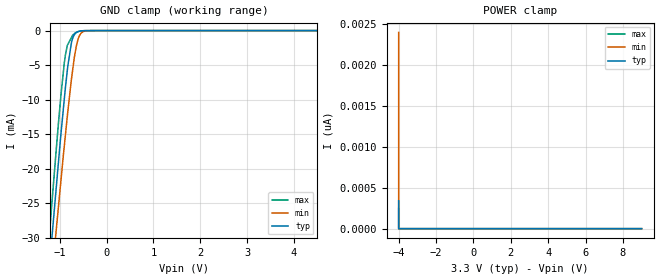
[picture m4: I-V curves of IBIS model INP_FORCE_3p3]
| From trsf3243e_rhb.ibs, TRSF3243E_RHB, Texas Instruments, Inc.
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[Model]   INP_FORCE_3p3
Model_type   Input
Vinl = 0.6
Vinh = 2.4
|   typ   min   max
C_comp   0.802pF	0.773pF	0.843pF
[Voltage Range]   3.3   3   3.6
[Temperature Range]   27   110   -40
[Power Clamp Reference]   3.3   3   3.6
[GND Clamp Reference]   0   0   0
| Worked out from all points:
|   GND clamp passes 1 mA (typ) near -0.72 V on its own axis
[GND Clamp]
|   Voltage   I(typ)   I(min)   I(max)
-4V       -268.4mA   -254.7mA   -282.4mA
-1.226V   -34.73mA   -40.07mA   -30.27mA
-1.166V   -30.07mA   -35.67mA   -25.03mA
-1.121V   -26.57mA   -32.35mA   -21.31mA
-1.038V   -20.04mA   -26.39mA   -14.37mA
-974mV    -15.1mA    -21.84mA   -9.461mA
-877.3mV  -8.272mA   -15.15mA   -3.53mA
-747.7mV  -1.719mA   -7.003mA   -998.5uA
-687.2mV  -601.2uA   -3.902mA   -457.1uA
-608.7mV  -166.4uA   -1.294mA   -144.1uA
-398.1mV  -10.92uA   -15.53uA   -3.434uA
9V        0A         0A         0A
[POWER Clamp]
|   Voltage   I(typ)   I(min)   I(max)
-4V       340.5pA    2.399nA    246.8pA
-4V       0A         0A         0A
-4V       0A         0A         0A
9V        0A         0A         0A
